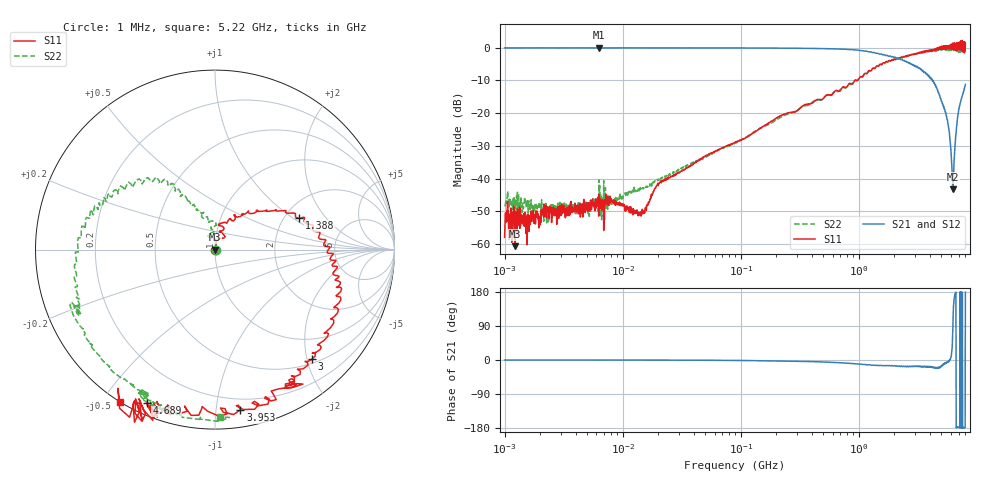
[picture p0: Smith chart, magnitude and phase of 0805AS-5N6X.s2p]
!s-Parameter Generated by FASTRON Sdn. Bhd.
!FASTRON P/N : 0805AS-5N6X
!Keysight Technologies: E5071C_MY46733604_B.14.02
!Date: Mon Jun 15 12:47:18 2026
!Version  :Rev01  Mon Jun 15 12:47:18 2026
!Data & Calibration Information:
!Freq  S11:SOLT2(ON)  S21:SOLT2(ON)  S12:SOLT2(ON)  S22:SOLT2(ON)
!PortZ  Port1:50+j0  Port2:50+j0
!When reading reference impedance value at option line is always used.
! Remarks : This data is being provided solely for informational purposes.
# Hz S dB R 50
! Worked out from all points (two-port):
!   1601 points, 1 MHz to 8 GHz, reference 50 ohm
!   highest |S21| = -0.01 dB at 6.301 MHz (marker M1); lowest = -43.3 dB at 6.265 GHz (marker M2)
!   |S21| within 3 dB of the highest: start of sweep to 2.057 GHz
!   lowest |S11| = -60.7 dB at 1.231 MHz (marker M3), VSWR 1.00, Z = 50.1 - j0.0099 ohm
!   |S11| at or under -10 dB: start of sweep to 922.7 MHz; 963 MHz to 974.2 MHz (11.23 MHz wide, 1.16 % of centre)
!   |S22| runs from -53.6 to -0.2 dB; largest |S21 - S12| = 0.0083
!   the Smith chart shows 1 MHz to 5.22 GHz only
!   S11 on the Smith chart (normalised r, x): 1 MHz: 1.00, -0.00; 1.388 GHz: 2.39, +1.12; 3 GHz: 0.57, -2.09; 3.953 GHz: 0.12, -1.16; 4.689 GHz: 0.05, -0.65; 5.22 GHz: -0.00, -0.55
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1000000  -58.00 -14.7  -0.04 -0.1  -0.03 -0.1  -48.50 5.9
1231028  -60.70 -6.2  -0.03 -0.0  -0.04 -0.0  -48.10 -2.7
2173433  -48.60 27.4  -0.03 -0.1  -0.03 -0.0  -50.30 35.3
4479405  -49.60 20.1  -0.04 -0.1  -0.04 -0.1  -49.60 29.2
6301378  -44.80 33.6  -0.01 -0.3  -0.01 -0.0  -40.40 39.7
1.414737e7  -50.20 58.8  -0.03 -0.2  -0.05 -0.3  -43.00 44.5
2.00676e7  -41.60 58.6  -0.04 -0.3  -0.05 -0.3  -40.40 65.4
8.994653e7  -28.90 78.8  -0.06 -1.2  -0.07 -1.2  -29.10 80.7
4.006501e8  -17.00 81.7  -0.20 -4.3  -0.20 -4.3  -16.80 87.7
1.388219e9  -6.03 20.6  -1.64 -14.5  -1.65 -14.6  -5.90 129.0
1.7949e9  -3.98 1.5  -2.61 -14.8  -2.61 -15.1  -3.95 146.0
2.472225e9  -2.67 -20.8  -4.20 -16.9  -4.26 -17.0  -2.63 166.0
3.000426e9  -1.77 -48.5  -5.42 -16.4  -5.46 -16.3  -2.01 -166.0
3.60885e9  -1.38 -65.4  -7.49 -18.1  -7.45 -17.9  -1.25 -151.0
3.95342e9  -0.88 -81.0  -8.78 -16.9  -8.77 -17.1  -1.13 -137.0
4.688537e9  -0.56 -114.0  -13.40 -21.9  -13.40 -22.1  -0.77 -113.0
5.220382e9  0.03 -122.0  -18.00 -10.0  -18.00 -10.5  -0.61 -88.2
5.64026e9  0.64 -140.0  -22.10 -5.8  -22.20 -5.9  -0.54 -60.8
6.265031e9  -0.42 -142.0  -43.30 84.2  -43.30 84.5  -0.47 -31.7
6.457806e9  -0.09 -145.0  -33.10 165.0  -32.90 165.0  -0.43 -17.3
7.036128e9  0.64 -168.0  -18.70 -178.0  -18.90 -178.0  -0.66 16.6
8e9  1.60 154.0  -11.20 179.0  -11.10 178.0  -0.81 43.4
